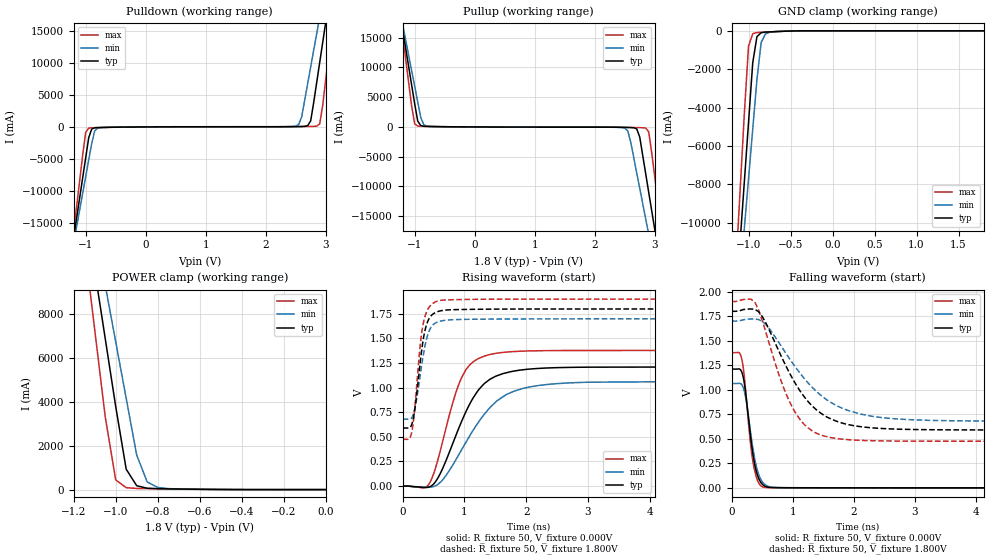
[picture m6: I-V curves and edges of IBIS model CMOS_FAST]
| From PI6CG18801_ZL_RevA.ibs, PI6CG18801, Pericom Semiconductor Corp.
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[Model]   CMOS_FAST
Model_type Output
Vref=1.800V
Vmeas=900mV
| variable   typ   min   max
C_comp   1.500pF   1.470pF   1.530pF
[Voltage Range]   1.8000V   1.7000V   1.9000V
[POWER Clamp Reference]   1.8000V   1.7000V   1.9000V
[GND Clamp Reference]   0.0000V   0.0000V   0.0000V
[Pullup Reference]   1.8000V   1.7000V   1.9000V
[Pulldown Reference]   0.0000V   0.0000V   0.0000V
[Temperature Range]   25   85   -40
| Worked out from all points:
|   slope of the pulldown table from 0 to 0.27 V, typ, clamps not added: 17.5 ohm
|   slope of the pullup table from 0 to 0.27 V, typ, clamps not added: 20 ohm
|   GND clamp passes 1 mA (typ) near -0.36 V on its own axis
|   POWER clamp passes 1 mA (typ) near -0.37 V on its own axis
|   falling waveform, R_fixture 50, V_fixture 0.000V: 20-80 % time 147ps typ, 159ps min, 134ps max; typ from 1.21 V to 0 V
|   rising waveform, R_fixture 50, V_fixture 0.000V: 20-80 % time 527ps typ, 692ps min, 381ps max; typ from 0 V to 1.21 V
|   falling waveform, R_fixture 50, V_fixture 1.800V: 20-80 % time 671ps typ, 835ps min, 506ps max; typ from 1.8 V to 0.59 V
|   rising waveform, R_fixture 50, V_fixture 1.800V: 20-80 % time 146ps typ, 162ps min, 131ps max; typ from 0.59 V to 1.8 V
[GND Clamp]
| Voltage   I(typ)   I(min)   I(max)
-1.8V     -54.4A     -49.03A    -63.81A
-1.15V    -14.07A    -15.45A    -12.25A
-1.1V     -10.97A    -12.87A    -8.279A
-1.05V    -7.863A    -10.28A    -4.312A
-1V       -4.761A    -7.702A    -788.1mA
-950mV    -1.659A    -5.119A    -151.5mA
-900mV    -303.5mA   -2.537A    -89.47mA
-850mV    -101.7mA   -613.1mA   -76.41mA
-800mV    -67.15mA   -167.4mA   -67.68mA
-750mV    -55.39mA   -73.22mA   -57.6mA
-350mV    -802.5uA   -1.671mA   -102.1uA
1.8V      15.03uA    17.5uA     13.92uA
[Power Clamp]
| Voltage   I(typ)   I(min)   I(max)
-1.8V     53.55A     48.18A     62.95A
-1.15V    13.12A     14.51A     11.28A
-1.1V     10.01A     11.92A     7.303A
-1.05V    6.902A     9.336A     3.331A
-1V       3.795A     6.749A     443mA
-950mV    930.5mA    4.162A     88.83mA
-900mV    176.9mA    1.578A     52.93mA
-850mV    63.4mA     349.1mA    44.07mA
-800mV    41.98mA    99.84mA    37.38mA
-750mV    33.29mA    45.32mA    30.27mA
-650mV    20.34mA    21.99mA    16.82mA
0V        15.03uA    15.03uA    14.69uA
[Pulldown]
| Voltage   I(typ)   I(min)   I(max)
-1.8V     -54.42A    -49.05A    -63.84A
-1.2V     -17.2A     -18.06A    -16.25A
-1V       -4.79A     -7.726A    -827.2mA
-950mV    -1.689A    -5.144A    -191.1mA
-750mV    -87.68mA   -99.6mA    -100.8mA
2.55V     59.88mA    370.4mA    52.99mA
2.75V     956.7mA    9.357A     80.67mA
2.85V     6.928A     14.53A     125.7mA
2.9V      10.03A     17.12A     480mA
3V        16.25A     22.3A      7.34A
3.1V      22.47A     27.48A     15.29A
3.6V      53.58A     53.39A     55.04A
[Pullup]
| Voltage   I(typ)   I(min)   I(max)
-1.8V     53.63A     48.25A     63.06A
-1.2V     16.29A     17.15A     15.33A
-1.05V    6.959A     9.386A     3.404A
-950mV    984.1mA    4.208A     156.8mA
-800mV    86.58mA    137.9mA    94.43mA
2.5V      -78.71mA   -194.9mA   -67.08mA
2.7V      -336.9mA   -7.729A    -111.4mA
2.85V     -7.897A    -15.48A    -195.5mA
2.9V      -11A       -18.06A    -832.2mA
3V        -17.2A     -23.23A    -8.323A
3.1V      -23.41A    -28.39A    -16.26A
3.6V      -54.44A    -54.22A    -55.93A
[Falling Waveform]
R_fixture = 50
V_fixture = 0.000V
V_fixture_min = 0.000V
V_fixture_max = 0.000V
|   Time   V(typ)   V(min)   V(max)
0s        1.211V     1.064V     1.378V
120ps     1.212V     1.065V     1.378V
156ps     1.192V     1.058V     1.334V
192ps     1.117V     1.016V     1.209V
228ps     968.1mV    919.6mV    988.9mV
300ps     566.3mV    606mV      495.4mV
348ps     338mV      399mV      262.2mV
432ps     111mV      151.9mV    62.65mV
552ps     14.22mV    30.32mV    4.12mV
20ns      8.648uV    9.578uV    8.14uV
[Rising Waveform]
R_fixture = 50
V_fixture = 0.000V
V_fixture_min = 0.000V
V_fixture_max = 0.000V
|   Time   V(typ)   V(min)   V(max)
0s        8.686uV    9.598uV    8.159uV
425ps     -9.398mV   -12.2mV    20.49mV
600ps     117.2mV    33.92mV    338.6mV
825ps     456.7mV    229.6mV    877.6mV
975ps     688.7mV    392.7mV    1.127V
1.225ns   976.2mV    647.9mV    1.296V
1.6ns     1.138V     897.9mV    1.357V
2.1ns     1.191V     1.012V     1.374V
3ns       1.208V     1.055V     1.378V
20ns      1.211V     1.064V     1.378V
[Falling Waveform]
R_fixture = 50
V_fixture = 1.800V
V_fixture_min = 1.700V
V_fixture_max = 1.900V
|   Time   V(typ)   V(min)   V(max)
0s        1.8V       1.7V       1.9V
375ps     1.82V      1.721V     1.896V
562.5ps   1.676V     1.663V     1.578V
875ps     1.258V     1.383V     980.8mV
1.125ns   981.9mV    1.163V     691.1mV
1.375ns   801.8mV    990mV      560.1mV
1.75ns    671.2mV    828.7mV    500.4mV
2.375ns   608.5mV    722.8mV    479.6mV
3.625ns   591.3mV    683.9mV    475.3mV
20ns      589.8mV    679.5mV    475mV
[Rising Waveform]
R_fixture = 50
V_fixture = 1.800V
V_fixture_min = 1.700V
V_fixture_max = 1.900V
|   Time   V(typ)   V(min)   V(max)
0s        589.8mV    679.5mV    475mV
110ps     591.9mV    679.6mV    483.2mV
150ps     633mV      698.7mV    559.8mV
200ps     800mV      799.9mV    825.2mV
290ps     1.294V     1.156V     1.472V
330ps     1.481V     1.319V     1.646V
360ps     1.581V     1.423V     1.723V
460ps     1.731V     1.615V     1.841V
650ps     1.785V     1.681V     1.89V
20ns      1.8V       1.7V       1.9V
[Ramp]
| variable   typ   min   max
dV/dt_r   0.72636V/525.56p   0.63822V/689.18p   0.82704V/380.57p
dV/dt_f   0.72594V/699.92p   0.61206V/830.60p   0.85482V/502.85p
R_load = 50
